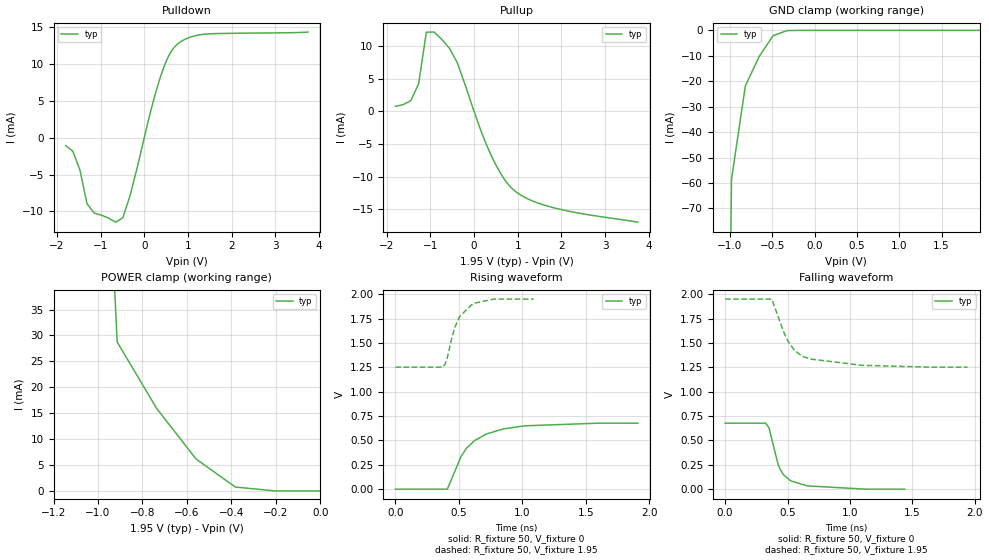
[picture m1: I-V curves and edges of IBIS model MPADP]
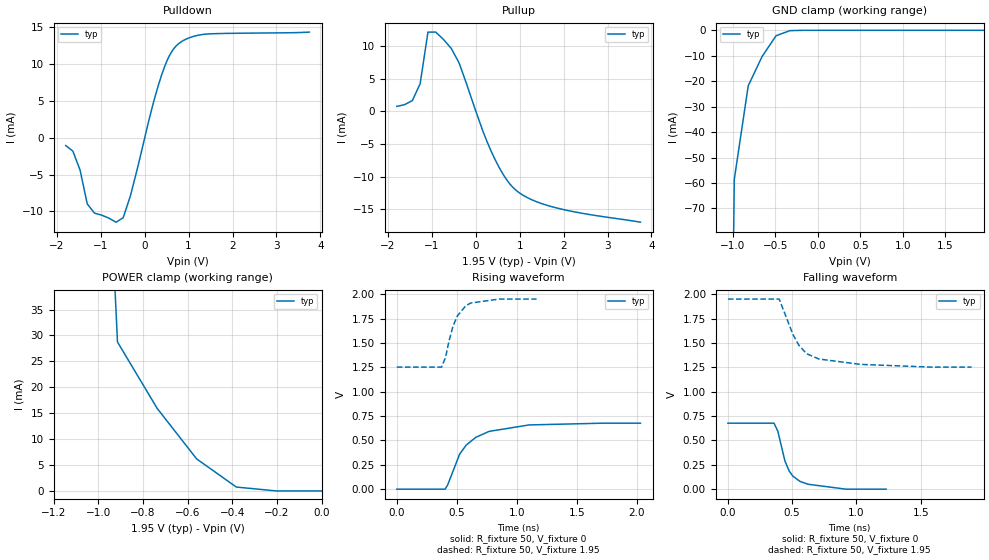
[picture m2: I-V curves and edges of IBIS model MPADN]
| Created by SiliconSmart 2008.10 (Production)
| There are several IBIS sections which it is inappropriate for this tool to
| automatically fill in - copyrights and packaging details are two examples.
| We are making it easy for you to add these things by providing commented-out
| section headers and brief descriptions of each such section.  Of course, the
| IBIS standard is the ultimate section description; these are merely summaries.
[IBIS Ver]   4.1
[File Name]   ff_1p32_1p95_m40c.ibs
[File Rev]   1.0
[Date]   December 18 11:22:01
[Source]   From SiliconSmart 2008.10 (Production)
|[Notes]   Use this section for any special notes related to the file.
|   (fill in and uncomment to use this section)
|[Disclaimer]   Legal disclaimer section.
|   (fill in and uncomment to use this section)
|[Copyright]   Copyright 1995, XYZ Corp., All Rights Reserved
|   (fill in and uncomment to use this section)
[Component]   pdqs_ddr2_cl_driver_6p9ma
[Manufacturer]   Unknown
[Package]
| Variable   typ   min   max
R_pkg   18   NA   NA
L_pkg   1n   NA   NA
C_pkg   15f   NA   NA
[Pin]   signal_name   model_name   R_pin   L_pin   C_pin
1   PADP   MPADP   NA   NA   NA
2   PADN   MPADN   NA   NA   NA
3   DVSS   GND   NA   NA   NA
4   DVDD   POWER   NA   NA   NA
|[Package Model]   Package model name.  40-char limit.
|   (fill in and uncomment to use this section)
[Pin Mapping]  pulldown_ref   pullup_ref   gnd_clamp_ref  power_clamp_ref
1   DVSS   DVDD   DVSS   DVDD
2   DVSS   DVDD   DVSS   DVDD
3   DVSS   NC   NC   NC
4   NC   DVDD   NC   NC
[Diff Pin]  inv_pin  vdiff  tdelay_typ tdelay_min tdelay_max
1   2   NA   -48.59p   NA   NA
| Models and submodels in the file (2): MPADP (I/O), MPADN (I/O)
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|PADP pin
[Model]   MPADP
Model_type I/O
Polarity Non-Inverting
Vinl = 0.8
Vinh = 2.0
Vmeas = 0.9
| Capacitance   typ   min   max
C_comp   6.42p   NA   NA
| Variables   typ   min   max
[Temperature Range]   -40   NA   NA
[Voltage Range]   1.95   NA   NA
[Pullup Reference]   1.95   NA   NA
[Pulldown Reference]   0.0   NA   NA
[POWER Clamp Reference]   1.95   NA   NA
[GND Clamp Reference]   0.0   NA   NA
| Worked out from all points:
|   slope of the pulldown table from 0 to 0.292 V, typ, clamps not added: 43.3 ohm
|   slope of the pullup table from 0 to 0.292 V, typ, clamps not added: 55.7 ohm
|   GND clamp passes 1 mA (typ) near -0.40 V on its own axis
|   POWER clamp passes 1 mA (typ) near -0.39 V on its own axis
|   falling waveform, R_fixture 50, V_fixture 0: 20-80 % time 110ps typ, NA min, NA max; typ from 0.677 V to 0 V
|   falling waveform, R_fixture 50, V_fixture 1.95: 20-80 % time 175ps typ, NA min, NA max; typ from 1.95 V to 1.25 V
|   rising waveform, R_fixture 50, V_fixture 0: 20-80 % time 231ps typ, NA min, NA max; typ from 0 V to 0.677 V
|   rising waveform, R_fixture 50, V_fixture 1.95: 20-80 % time 120ps typ, NA min, NA max; typ from 1.25 V to 1.95 V
[Pulldown]
| Voltage   I(typ)   I(min)   I(max)
-1.8V     -1.059mA   NA         NA
-1.636V   -1.817mA   NA         NA
-1.473V   -4.395mA   NA         NA
-1.309V   -8.977mA   NA         NA
-654.5mV  -11.46mA   NA         NA
-490.9mV  -10.86mA   NA         NA
-327.3mV  -7.893mA   NA         NA
337.5mV   7.644mA    NA         NA
534.4mV   10.81mA    NA         NA
731.2mV   12.56mA    NA         NA
1.378V    14.06mA    NA         NA
3.75V     14.35mA    NA         NA
[GND Clamp]
| Voltage   I(typ)   I(min)   I(max)
-1.8V     -4.304A    NA         NA
-1.145V   -514.4mA   NA         NA
-981.8mV  -58.54mA   NA         NA
-818.2mV  -21.8mA    NA         NA
-654.5mV  -10.26mA   NA         NA
-490.9mV  -2.127mA   NA         NA
-327.3mV  -116.5uA   NA         NA
1.95V     14.04nA    NA         NA
[Pullup]
| Voltage   I(typ)   I(min)   I(max)
-1.8V     761.5uA    NA         NA
-1.445V   1.656mA    NA         NA
-1.268V   4.237mA    NA         NA
-1.091V   12.14mA    NA         NA
-913.6mV  12.14mA    NA         NA
-559.1mV  9.631mA    NA         NA
-381.8mV  7.428mA    NA         NA
318.7mV   -5.636mA   NA         NA
628.1mV   -9.711mA   NA         NA
881.2mV   -11.88mA   NA         NA
1.781V    -14.7mA    NA         NA
3.75V     -16.98mA   NA         NA
[POWER Clamp]
| Voltage   I(typ)   I(min)   I(max)
-1.8V     4.305A     NA         NA
-1.623V   3.15A      NA         NA
-1.445V   2.032A     NA         NA
-1.268V   990.8mA    NA         NA
-1.091V   190.7mA    NA         NA
-913.6mV  28.75mA    NA         NA
-736.4mV  15.95mA    NA         NA
-559.1mV  6.178mA    NA         NA
-381.8mV  749.4uA    NA         NA
-204.5mV  4.037uA    NA         NA
-27.27mV  14.87nA    NA         NA
0V        0A         NA         NA
[Ramp]
dV/dt_r   0.412458/0.175423n NA   NA
dV/dt_f   0.412465/0.142654n NA   NA
R_load = 50
[Falling Waveform]
R_fixture = 50
V_fixture = 0
| Time   V(typ)   V(min)   V(max)
0s        676.9mV    NA         NA
324.2ps   676.9mV    NA         NA
350.7ps   632mV      NA         NA
423.7ps   256.5mV    NA         NA
440.5ps   205.2mV    NA         NA
469.4ps   145.6mV    NA         NA
524.1ps   85.92mV    NA         NA
657.3ps   33.64mV    NA         NA
1.127ns   21.07uV    NA         NA
1.439ns   21.07uV    NA         NA
[Falling Waveform]
R_fixture = 50
V_fixture = 1.95
| Time   V(typ)   V(min)   V(max)
0s        1.95V      NA         NA
374.1ps   1.95V      NA         NA
468.6ps   1.613V     NA         NA
504.9ps   1.515V     NA         NA
555.7ps   1.424V     NA         NA
615.8ps   1.364V     NA         NA
678.1ps   1.336V     NA         NA
1.099ns   1.27V      NA         NA
1.631ns   1.252V     NA         NA
1.943ns   1.252V     NA         NA
[Rising Waveform]
R_fixture = 50
V_fixture = 0
| Time   V(typ)   V(min)   V(max)
0s        21.3uV     NA         NA
409.1ps   21.3uV     NA         NA
518.4ps   339mV      NA         NA
560.4ps   420.1mV    NA         NA
622.5ps   497.4mV    NA         NA
716.4ps   565.6mV    NA         NA
849.3ps   617.8mV    NA         NA
1.019ns   649.9mV    NA         NA
1.597ns   676.9mV    NA         NA
1.91ns    676.9mV    NA         NA
[Rising Waveform]
R_fixture = 50
V_fixture = 1.95
| Time   V(typ)   V(min)   V(max)
0s        1.252V     NA         NA
373.6ps   1.252V     NA         NA
390.1ps   1.279V     NA         NA
408ps     1.343V     NA         NA
443.1ps   1.544V     NA         NA
470.4ps   1.666V     NA         NA
506.1ps   1.772V     NA         NA
612.5ps   1.905V     NA         NA
776.8ps   1.95V      NA         NA
1.089ns   1.95V      NA         NA
|PADN pin
[Model]   MPADN
Model_type I/O
Polarity Inverting
Vinl = 0.8
Vinh = 2.0
Vmeas = 0.9
| Capacitance   typ   min   max
C_comp   6.42p   NA   NA
| Variables   typ   min   max
[Temperature Range]   -40   NA   NA
[Voltage Range]   1.95   NA   NA
[Pullup Reference]   1.95   NA   NA
[Pulldown Reference]   0.0   NA   NA
[POWER Clamp Reference]   1.95   NA   NA
[GND Clamp Reference]   0.0   NA   NA
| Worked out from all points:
|   slope of the pulldown table from 0 to 0.292 V, typ, clamps not added: 43.3 ohm
|   slope of the pullup table from 0 to 0.292 V, typ, clamps not added: 55.7 ohm
|   GND clamp passes 1 mA (typ) near -0.40 V on its own axis
|   POWER clamp passes 1 mA (typ) near -0.39 V on its own axis
|   falling waveform, R_fixture 50, V_fixture 0: 20-80 % time 107ps typ, NA min, NA max; typ from 0.677 V to 0 V
|   falling waveform, R_fixture 50, V_fixture 1.95: 20-80 % time 171ps typ, NA min, NA max; typ from 1.95 V to 1.25 V
|   rising waveform, R_fixture 50, V_fixture 0: 20-80 % time 224ps typ, NA min, NA max; typ from 0 V to 0.677 V
|   rising waveform, R_fixture 50, V_fixture 1.95: 20-80 % time 114ps typ, NA min, NA max; typ from 1.25 V to 1.95 V
[Pulldown]
| Voltage   I(typ)   I(min)   I(max)
-1.8V     -1.059mA   NA         NA
-1.636V   -1.817mA   NA         NA
-1.473V   -4.395mA   NA         NA
-1.309V   -8.977mA   NA         NA
-654.5mV  -11.46mA   NA         NA
-490.9mV  -10.86mA   NA         NA
-327.3mV  -7.893mA   NA         NA
337.5mV   7.644mA    NA         NA
534.4mV   10.81mA    NA         NA
731.2mV   12.56mA    NA         NA
1.378V    14.06mA    NA         NA
3.75V     14.35mA    NA         NA
[GND Clamp]
| Voltage   I(typ)   I(min)   I(max)
-1.8V     -4.304A    NA         NA
-1.145V   -514.4mA   NA         NA
-981.8mV  -58.54mA   NA         NA
-818.2mV  -21.8mA    NA         NA
-654.5mV  -10.26mA   NA         NA
-490.9mV  -2.127mA   NA         NA
-327.3mV  -116.5uA   NA         NA
1.95V     14.04nA    NA         NA
[Pullup]
| Voltage   I(typ)   I(min)   I(max)
-1.8V     761.5uA    NA         NA
-1.445V   1.656mA    NA         NA
-1.268V   4.237mA    NA         NA
-1.091V   12.14mA    NA         NA
-913.6mV  12.14mA    NA         NA
-559.1mV  9.631mA    NA         NA
-381.8mV  7.428mA    NA         NA
318.7mV   -5.636mA   NA         NA
628.1mV   -9.711mA   NA         NA
881.2mV   -11.88mA   NA         NA
1.781V    -14.7mA    NA         NA
3.75V     -16.98mA   NA         NA
[POWER Clamp]
| Voltage   I(typ)   I(min)   I(max)
-1.8V     4.305A     NA         NA
-1.623V   3.15A      NA         NA
-1.445V   2.032A     NA         NA
-1.268V   990.8mA    NA         NA
-1.091V   190.7mA    NA         NA
-913.6mV  28.75mA    NA         NA
-736.4mV  15.95mA    NA         NA
-559.1mV  6.178mA    NA         NA
-381.8mV  749.4uA    NA         NA
-204.5mV  4.037uA    NA         NA
-27.27mV  14.87nA    NA         NA
0V        0A         NA         NA
[Ramp]
dV/dt_r   0.412458/0.168814n NA   NA
dV/dt_f   0.412465/0.138942n NA   NA
R_load = 50
[Falling Waveform]
R_fixture = 50
V_fixture = 0
| Time   V(typ)   V(min)   V(max)
0s        676.9mV    NA         NA
358.7ps   676.9mV    NA         NA
388.2ps   594.9mV    NA         NA
443.4ps   290.4mV    NA         NA
476.3ps   186.9mV    NA         NA
506.4ps   132.5mV    NA         NA
560.4ps   80.22mV    NA         NA
622.5ps   50.65mV    NA         NA
918.4ps   21.19uV    NA         NA
1.231ns   21.19uV    NA         NA
[Falling Waveform]
R_fixture = 50
V_fixture = 1.95
| Time   V(typ)   V(min)   V(max)
0s        1.95V      NA         NA
399ps     1.95V      NA         NA
506.1ps   1.586V     NA         NA
552.9ps   1.475V     NA         NA
612.5ps   1.39V      NA         NA
707.3ps   1.335V     NA         NA
1.033ns   1.28V      NA         NA
1.583ns   1.252V     NA         NA
1.896ns   1.252V     NA         NA
[Rising Waveform]
R_fixture = 50
V_fixture = 0
| Time   V(typ)   V(min)   V(max)
0s        20.89uV    NA         NA
402.7ps   20.89uV    NA         NA
423.7ps   43mV       NA         NA
524.1ps   360.8mV    NA         NA
579.2ps   453mV      NA         NA
657.3ps   530.9mV    NA         NA
769.2ps   592.6mV    NA         NA
1.102ns   658.8mV    NA         NA
1.718ns   676.9mV    NA         NA
2.031ns   676.9mV    NA         NA
[Rising Waveform]
R_fixture = 50
V_fixture = 1.95
| Time   V(typ)   V(min)   V(max)
0s        1.252V     NA         NA
372.3ps   1.252V     NA         NA
405.8ps   1.35V      NA         NA
433.4ps   1.511V     NA         NA
468.6ps   1.673V     NA         NA
505ps     1.778V     NA         NA
574.6ps   1.881V     NA         NA
615.8ps   1.909V     NA         NA
852.4ps   1.95V      NA         NA
1.165ns   1.95V      NA         NA
